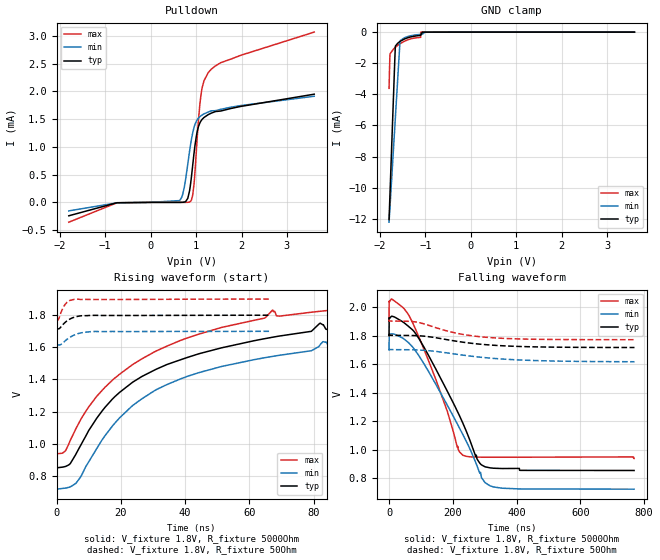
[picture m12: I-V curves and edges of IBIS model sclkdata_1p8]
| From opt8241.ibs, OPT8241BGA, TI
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|   sclkdata_1p8 Model
[Model]   sclkdata_1p8
Model_type   I/O_open_drain
Polarity   Inverting
Vinl = 0.54
Vinh = 1.26
Vmeas = 0.9
Vref = 1.8
Cref = 2pF
Rref = 20000
|   typ   min   max
|   (nom PVT)   (fast PVT)   (slow PVT)
C_comp   3.942e-13   2.845e-13   5.249e-13
[Model spec]
|subparameter
Vinl   0.54   0.51   0.57
Vinh   1.26   1.19   1.33
| Where nom  PVT is Nominal Process, 1.8V, 27C
|   Fast PVT is Strong Process,  1.9V, -40C
|   Slow PVT is Weak Process,   1.7V, 125C
[Voltage Range]   1.8   1.7   1.9
|Junction Temperature
[Temperature Range]   27   125   -40
[Pullup Reference]   1.8   1.7   1.9
[Pulldown Reference]   0   0   0
[Power Clamp Reference]   1.8   1.7   1.9
[GND Clamp Reference]   0   0   0
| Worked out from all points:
|   GND clamp passes 1 mA (typ) near -1.66 V on its own axis
|   falling waveform, V_fixture 1.8V, R_fixture 5000Ohm: 20-80 % time 122ns typ, 135ns min, 92.2ns max; typ from 1.8 V to 0.853 V
|   rising waveform, V_fixture 1.8V, R_fixture 5000Ohm: 20-80 % time 45.5ns typ, 45.9ns min, 41.6ns max; typ from 0.853 V to 1.8 V
|   falling waveform, V_fixture 1.8V, R_fixture 50Ohm: 20-80 % time 171ns typ, 207ns min, 145ns max; typ from 1.8 V to 1.72 V
|   rising waveform, V_fixture 1.8V, R_fixture 50Ohm: 20-80 % time 3.32ns typ, 4.07ns min, 1.96ns max; typ from 1.72 V to 1.8 V
[Pulldown]
|   Voltage   I(typ)   I(min)   I(max)
-1.8V     -241.6uA   -153.6uA   -357uA
-747.4mV  -7.723uA   -8.571uA   -9.083uA
639.5mV   114.7nA    32.63uA    107.3pA
741.5mV   5.307uA    272.4uA    25.63nA
817.2mV   71.68uA    686.9uA    1.019uA
872.4mV   290.1uA    1.006mA    14.22uA
955mV     884.1uA    1.349mA    328.4uA
1.055V    1.371mA    1.521mA    1.504mA
1.114V    1.475mA    1.564mA    1.969mA
1.268V    1.582mA    1.629mA    2.339mA
1.546V    1.647mA    1.678mA    2.519mA
3.6V      1.95mA     1.913mA    3.069mA
[GND Clamp]
|   Voltage   I(typ)   I(min)   I(max)
-1.8V     -12.05mA   -12.22mA   -3.615mA
-1.785V   -10.82mA   -11.49mA   -1.844mA
-1.777V   -10.2mA    -11.12mA   -1.394mA
-1.663V   -1.013mA   -5.609mA   -982.9uA
-1.567V   -619.4uA   -963.9uA   -763.1uA
-1.559V   -601.9uA   -613.6uA   -746.7uA
-1.552V   -588uA     -538.3uA   -733.6uA
-1.105V   -205.1uA   -142.6uA   -336.5uA
-1.103V   -204.3uA   -142uA     -5.373uA
-1.069V   -6.612uA   -133uA     -3.317uA
-1.006V   -3.129uA   -10.63uA   -1.251uA
3.6V      0A         0A         0A
[POWER Clamp]
|   Voltage   I(typ)   I(min)   I(max)
-1.8V     0A         0A         0A
0V        0A         0A         0A
3.6V      0A         0A         0A
[Ramp]
R_load = 5000
|   typ   min   max
dV/dt_r   0.567676/4.51892e-08   0.586127/4.54319e-08   0.577394/4.14964e-08
dV/dt_f   0.568146/1.21553e-07   0.586792/1.35379e-07   0.577742/9.22797e-08
[Falling Waveform]
V_fixture = 1.8V
V_fixture_min = 1.7V
V_fixture_max = 1.9V
R_fixture = 5000Ohm
|   Time   V(typ)   V(min)   V(max)
0s        1.8V       1.7V       1.9V
500ps     1.923V     1.797V     2.043V
7ns       1.934V     1.811V     2.056V
63.4ns    1.86V      1.745V     1.937V
147.2ns   1.563V     1.456V     1.49V
214.5ns   1.268V     1.179V     1.015V
231.8ns   1.184V     1.104V     959.6mV
279.7ns   920.9mV    863.2mV    946.7mV
317.5ns   871.4mV    744.7mV    946.1mV
769ns     853.1mV    722mV      937.4mV
[Rising Waveform]
V_fixture = 1.8V
V_fixture_min = 1.7V
V_fixture_max = 1.9V
R_fixture = 5000Ohm
|   Time   V(typ)   V(min)   V(max)
0s        853.1mV    722mV      937.1mV
2.7ns     859.2mV    725.2mV    955mV
6.1ns     939.2mV    756.4mV    1.097V
15.1ns    1.227V     1.051V     1.352V
26.5ns    1.418V     1.279V     1.528V
40.8ns    1.538V     1.42V      1.659V
67.2ns    1.663V     1.544V     1.831V
82.9ns    1.74V      1.635V     1.826V
164.1ns   1.78V      1.671V     1.895V
359.9ns   1.799V     1.699V     1.899V
[Falling Waveform]
V_fixture = 1.8V
V_fixture_min = 1.7V
V_fixture_max = 1.9V
R_fixture = 50Ohm
|   Time   V(typ)   V(min)   V(max)
0s        1.8V       1.7V       1.9V
200ps     1.806V     1.705V     1.909V
700ps     1.802V     1.703V     1.902V
84.5ns    1.799V     1.699V     1.895V
137.1ns   1.788V     1.691V     1.862V
212.4ns   1.76V      1.669V     1.816V
261.8ns   1.745V     1.654V     1.798V
321ns     1.733V     1.641V     1.785V
469.1ns   1.72V      1.624V     1.774V
770.2ns   1.716V     1.616V     1.771V
[Rising Waveform]
V_fixture = 1.8V
V_fixture_min = 1.7V
V_fixture_max = 1.9V
R_fixture = 50Ohm
|   Time   V(typ)   V(min)   V(max)
0s        1.716V     1.615V     1.771V
600ps     1.715V     1.615V     1.773V
1.3ns     1.725V     1.617V     1.812V
1.9ns     1.739V     1.626V     1.84V
3ns       1.76V      1.645V     1.874V
4ns       1.774V     1.66V      1.89V
5.6ns     1.787V     1.677V     1.898V
7.8ns     1.796V     1.69V      1.897V
11.9ns    1.799V     1.698V     1.897V
66.2ns    1.799V     1.699V     1.9V
